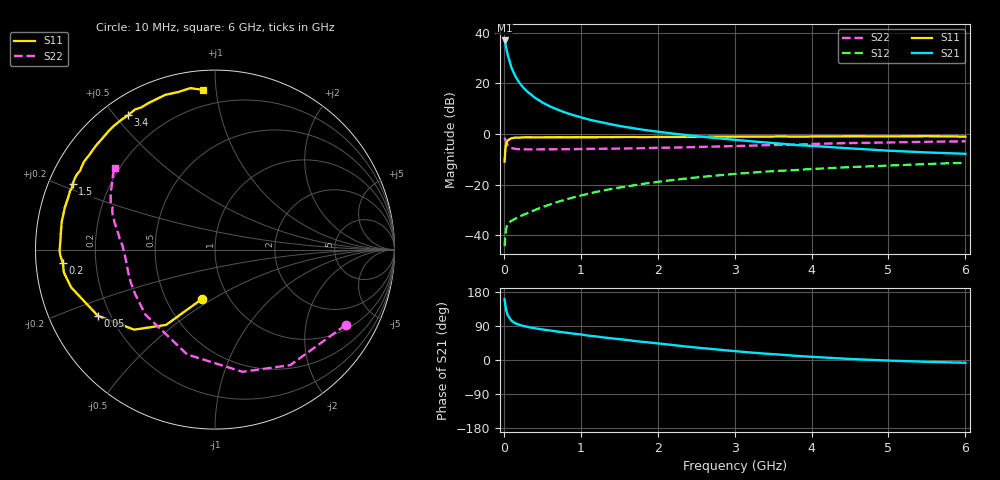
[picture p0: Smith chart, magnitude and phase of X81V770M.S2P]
! SIEMENS Small Signal Semiconductors
! BFP136W
! Si NPN RF Bipolar Junction Transistor in SOT343
! VCE = 1.75 V  IC = 70 mA
! Common Emitter S-Parameters:  September  1994
# GHz  S  MA  R  50
!  f  S11  S21  S12  S22
! GHz  MAG  ANG  MAG  ANG  MAG  ANG  MAG  ANG
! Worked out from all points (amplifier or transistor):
!   40 points, 10 MHz to 6 GHz, reference 50 ohm
!   highest |S21| = 37.0 dB at 10 MHz (marker M1)
!   |S21| within 3 dB of that: start of sweep to 31.59 MHz
!   unconditionally stable (mu >= 1): 526.7 MHz to 2.895 GHz
!   at 200 MHz: K = 0.65, MSG = 26.5 dB, |S12| = -32.6 dB
!   at 1.5 GHz: K = 1.10, MAG = 10.3 dB, |S12| = -21.1 dB
!   at 6 GHz: K = 0.98, MSG = 1.8 dB, |S12| = -11.3 dB
!   S11 on the Smith chart (normalised r, x): 10 MHz: 0.75, -0.45; 50 MHz: 0.15, -0.26; 200 MHz: 0.08, -0.04; 1.5 GHz: 0.07, +0.22; 3.4 GHz: 0.07, +0.54; 6 GHz: 0.11, +0.92
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0.01  0.2857 -105.0  70.84 160.4  0.0061 69.9  0.8411 -29.9
0.02  0.5004 -123.0  60.98 144.1  0.0106 57.7  0.7683 -56.9
0.03  0.634 -135.3  51.51 132.4  0.0136 48.3  0.6979 -77.3
0.05  0.75 -150.6  36.84 118.2  0.0168 38.4  0.6044 -104.9
0.1  0.8287 -165.3  20.41 103.5  0.0194 33.9  0.5306 -137.1
0.15  0.8514 -171.4  13.89 96.9  0.0213 36.2  0.5095 -150.6
0.2  0.8515 -175.0  10.42 93.0  0.0234 38.2  0.5038 -157.9
0.25  0.8626 -177.9  8.412 90.0  0.0252 41.5  0.5013 -162.4
0.3  0.8659 -179.6  7.031 87.8  0.0271 44.4  0.4992 -165.6
0.4  0.8628 176.7  5.293 83.9  0.0315 48.5  0.4991 -169.7
0.5  0.8638 174.0  4.22 80.6  0.036 52.1  0.4995 -172.5
0.6  0.8651 172.1  3.526 78.0  0.0406 54.5  0.5005 -174.2
0.7  0.8681 169.6  3.036 74.9  0.0457 57.0  0.502 -175.6
0.9  0.8677 166.3  2.377 69.7  0.0559 58.7  0.5046 -178.1
1.1  0.868 161.7  1.948 64.2  0.0663 59.7  0.5092 -179.7
1.5  0.874 155.2  1.451 55.0  0.0876 59.5  0.5173 177.2
2.2  0.8767 142.9  1.022 39.4  0.1237 54.8  0.5404 171.8
3.2  0.8916 125.9  0.724 19.9  0.1719 45.6  0.5897 162.9
3.4  0.8916 122.9  0.684 16.8  0.1815 43.5  0.6036 161.0
4.5  0.9058 107.9  0.522 2.7  0.2223 33.3  0.6646 150.9
5.5  0.9101 98.7  0.434 -4.8  0.2557 25.3  0.7046 143.8
6  0.8926 94.4  0.408 -7.3  0.2717 20.9  0.7198 140.7
